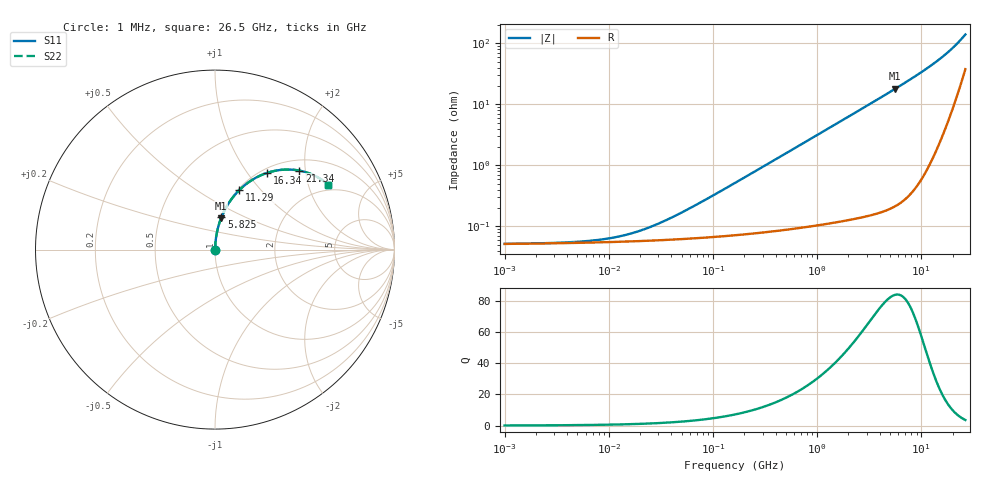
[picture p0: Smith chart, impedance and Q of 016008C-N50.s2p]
# MHz S MA R 50
!Freq  MagS11  AngS11  MagS21  AngS21  MagS12  AngS12  MagS22  AngS22
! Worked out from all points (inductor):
!   801 points, 1 MHz to 26.5 GHz, reference 50 ohm
!   read as one part in series: L = 500 pH near 61.08 MHz
!   highest Q = 84.1 at 5.607 GHz (marker M1), where L = 511 pH
!   S11 on the Smith chart (normalised r, x): 1 MHz: 1.00, +0.00; 5.825 GHz: 1.00, +0.37; 11.29 GHz: 1.02, +0.78; 16.34 GHz: 1.07, +1.24; 21.34 GHz: 1.23, +1.86; 26.5 GHz: 1.76, +2.70
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1  0.0005177 3.5  0.9995 -0.0  0.9995 -0.0  0.0005177 3.5
2.76901  0.0005351 9.3  0.9995 -0.0  0.9995 -0.0  0.0005351 9.3
5.506729  0.0005666 17.8  0.9995 -0.0  0.9995 -0.0  0.0005666 17.8
8.933011  0.0006178 27.0  0.9994 -0.0  0.9994 -0.0  0.0006178 27.0
13.42541  0.0007025 36.8  0.9994 -0.0  0.9994 -0.0  0.0007025 36.8
19.9218  0.00085 47.3  0.9994 -0.0  0.9994 -0.0  0.00085 47.3
29.94045  0.001111 57.7  0.9994 -0.1  0.9994 -0.1  0.001111 57.7
58.78931  0.00195 71.0  0.9994 -0.1  0.9994 -0.1  0.00195 71.0
162.7882  0.00516 81.7  0.9993 -0.3  0.9993 -0.3  0.00516 81.7
896.4305  0.02816 86.3  0.9986 -1.6  0.9986 -1.6  0.02816 86.3
2329.142  0.07316 84.8  0.996 -4.2  0.996 -4.2  0.07316 84.8
4873.952  0.1535 80.5  0.9863 -8.8  0.9863 -8.8  0.1535 80.5
5606.617  0.1768 79.1  0.9821 -10.2  0.9821 -10.2  0.1768 79.1
5824.894  0.1838 78.7  0.9808 -10.6  0.9808 -10.6  0.1838 78.7
8426.18  0.267 73.7  0.96 -15.5  0.96 -15.5  0.267 73.7
11292.73  0.3592 67.7  0.9255 -21.0  0.9255 -21.0  0.3592 67.7
13668.94  0.4346 62.4  0.8863 -25.7  0.8863 -25.7  0.4346 62.4
16335.85  0.5155 55.9  0.8295 -31.0  0.8295 -31.0  0.5155 55.9
18791.49  0.5836 49.7  0.7652 -35.6  0.7652 -35.6  0.5836 49.7
21342.82  0.6443 43.1  0.6882 -39.7  0.6882 -39.7  0.6443 43.1
25184.29  0.7109 33.2  0.5618 -43.9  0.5618 -43.9  0.7109 33.2
26500  0.7262 30.0  0.5187 -44.4  0.5187 -44.4  0.7262 30.0
